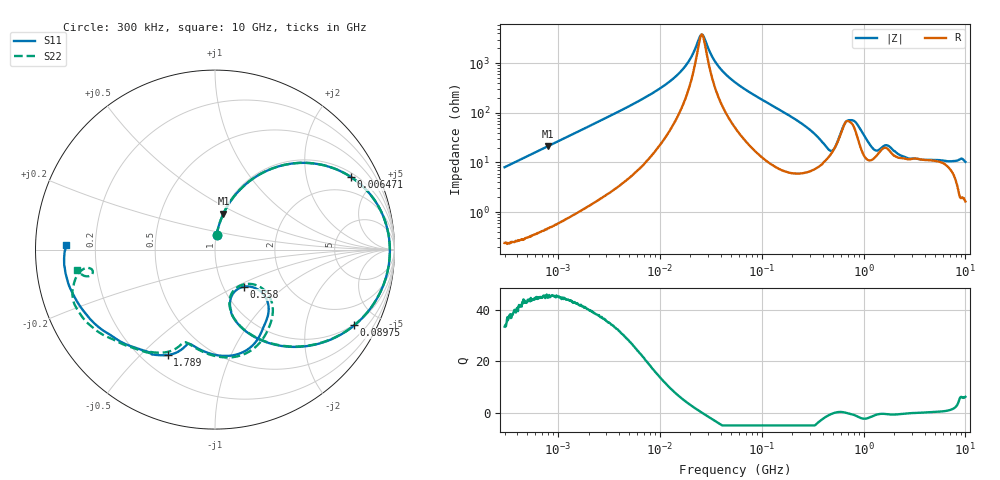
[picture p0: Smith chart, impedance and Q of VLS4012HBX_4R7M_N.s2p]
! S-Parameter Data Generated by TDK Corporation
! Copyright(C) 2023 TDK Corporation.
! All Rights Reserved.
! TDK P/N: VLS4012HBX-4R7M-N (Inductor)
! Property: L=4.7uH at 1MHz
! Size(LxWxT): 4x4x1.2mm
! Model Type: s2p (Touchstone File Format Version 1.0)
! Frequency: DC=Yes Start=0.3MHz Stop=10000MHz 802points Log-sweep
! Model Generated on June 16, 2023
! Port Assignments:
!  1 ---@@@--- 2
! Applicable Conditions:
!  Temperature = 25 degC
!  DC Bias Current = 0 A
!  Small Signal Operation
! Terms and conditions regarding TDK Simulation Models
! (1)This simulation model is being provided solely for informational purposes. Please refer to the specifications of the products in terms of detailed characteristics of such products.
! (2)In no event shall TDK Corporation of any of its subsidiaries be liable for any loss or damage arising, directly or indirectly,
!  From any information contained in this simulation model, including, but not limited to loss or damages arising from any inaccuracies, omissions or errors in connection with such information.
! (3)Any and all copyrights on this simulation model are owned by TDK Corporation.
!  Duplication or redistribution of this simulation model without prior written permission from TDK Corporation is prohibited.
! (4)This simulation model is subject to any modification or change without any prior notice.
! (5)Neither TDK Corporation nor any of its subsidiaries shall make any warranty, express or implied,
!  Including but not limited to the correctness, implied warranties of merchantability and fitness for a particular purpose with respect to this simulation models.
! (6)The use of this simulation model shall be deemed to have consented to the terms and conditions hereof.
# Hz S MA R 50
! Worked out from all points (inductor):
!   801 points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, 300 kHz to 10 GHz, reference 50 ohm
!   read as one part in series: L = 4.25 uH near 318.3 kHz
!   highest Q = 45.7 at 796.4 kHz (marker M1), where L = 4.24 uH
!   self-resonance near 25.9 MHz
!   S11 on the Smith chart (normalised r, x): 300 kHz: 1.00, +0.16; 6.471 MHz: 1.18, +3.64; 89.75 MHz: 0.96, -3.70; 558 MHz: 1.24, -0.55; 1.789 GHz: 0.30, -0.60; 10 GHz: 0.09, +0.02
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300000  0.07953 83.7  0.9944 -4.6  0.9945 -4.6  0.07932 83.7
796418  0.2063 76.8  0.9739 -12.0  0.9739 -12.0  0.2063 76.8
1713600  0.4102 64.3  0.9021 -24.3  0.9023 -24.3  0.4102 64.3
3509086  0.674 45.8  0.719 -42.5  0.7191 -42.5  0.674 45.8
6470506  0.859 28.1  0.4757 -59.4  0.4759 -59.4  0.859 28.1
9671944  0.9276 17.8  0.3151 -68.2  0.3151 -68.2  0.9278 17.8
1.740512e7  0.969 5.8  0.118 -72.4  0.1181 -72.4  0.9691 5.8
2.599165e7  0.9743 -1.4  0.02567 1.0  0.02568 1.0  0.9744 -1.3
3.642588e7  0.9687 -7.4  0.1016 67.5  0.1016 67.5  0.9688 -7.4
5.477226e7  0.9466 -15.8  0.2276 67.3  0.2277 67.3  0.9466 -15.7
8.974917e7  0.8835 -28.5  0.4088 57.4  0.4089 57.4  0.8834 -28.4
1.720721e8  0.7044 -50.3  0.6669 36.2  0.667 36.2  0.7043 -50.1
3.126428e8  0.465 -70.8  0.8283 12.1  0.8285 12.1  0.4647 -70.7
4.448526e8  0.3101 -74.4  0.8472 -4.5  0.8473 -4.5  0.3078 -74.9
5.580434e8  0.2611 -52.5  0.772 -18.7  0.7721 -18.7  0.2482 -52.0
7.152593e8  0.4903 -54.6  0.5453 -16.8  0.5454 -16.8  0.5063 -51.8
8.758105e8  0.5937 -75.7  0.6057 -6.8  0.6057 -6.9  0.6071 -76.9
1.10164e9  0.5693 -96.5  0.7214 -16.9  0.7215 -16.9  0.5692 -98.1
1.767019e9  0.6383 -113.4  0.6027 -39.9  0.6028 -39.9  0.6308 -115.2
1.788985e9  0.6439 -114.2  0.6006 -40.2  0.6007 -40.2  0.6367 -115.9
4.107799e9  0.8009 -152.6  0.3927 -74.7  0.3928 -74.7  0.8077 -147.4
1e10  0.8299 178.1  0.2225 -112.0  0.2226 -112.1  0.7755 -171.6
